FUNCTION_BLOCK FB_IEDClient IMPLEMENTS I_ScsmAbortIndEventSink, I_ScsmGetServerDirectoryCnfEventSink, I_ScsmGetLogicalDeviceDirectoryCnfEventSink, I_ScsmGetLogicalNodeDirectoryCnfEventSink, I_ScsmGetDataValuesCnfEventSink, I_ScsmSetDataValuesCnfEventSink, I_ScsmReportIndEventSink, I_ScsmControlCnfEventSink, I_ScsmLastApplErrorIndEventSink, I_ScsmCommandTerminationIndEventSink
VAR_INPUT
	fbConnection		: FB_iec61850ClientClass := (ipAbortInd:=THIS^, ipGetServerDirectoryCnf:=THIS^, ipGetLogicalDeviceDirectoryCnf:=THIS^, ipGetLogicalNodeDirectoryCnf:=THIS^, ipGetDataValuesCnf:=THIS^, ipSetDataValuesCnf:=THIS^, ipReportInd:=THIS^, ipControlCnf:=THIS^, ipLastApplErrorInd:=THIS^, ipCommandTerminationInd:=THIS^);
END_VAR
VAR
	_bAbort				: BOOL; (* Rising edge activates AbortReq() command execution *)
	_bDisconnect		: BOOL; (* Rising edge activates ReleaseReq() command execution *)
	_bConnect			: BOOL; (* Rising edge activates AssociateReq() command execution *)
	_bReconnect			: BOOL := TRUE; (* TRUE => reconnect automatically *)
	_bReadAllData		: BOOL := TRUE; (* TRUE => read/refresh all data values on reconnect *)
	
	state				: BYTE;
	eState				: E_AsyncEnvironmentState; (* Environment state *)
	bBusy				: BOOL; (* If TRUE => command execution is busy *)
	bSuccess			: BOOL;
	ipResult			: I_AsyncServiceResultClass;
	sLastErrorResult	: T_MaxString;
	fbAbortReason		: FB_ServiceErrorClass := (stError:=SUCCESS_EVENT);
	sLastAbortReason	: T_MaxString;
	nInvokeID			: UDINT;
	eServiceError		: E_AcsiServiceError; (* Latest OnXyzCnf() or OnXyzInd() event handler error *)
	nServiceError		: UDINT; (* Counts OnXyzCnf() and OnXyzInd() event handler errors *)
	nCmdError			: UDINT; (* Counts xyzReq() command errors *)
	sObjReference		: T_AcsiObjectReference; (* DATA object reference *)
	sCtrlReference		: T_AcsiObjectReference; (* CONTROLLABLE-DATA object reference *)
	
	bGetServerDirectory				: BOOL := TRUE; (* Rising edge enumerates logical-devices *)
	bGetLogicalDeviceDirectory		: BOOL := TRUE; (* Rising edge enumerates logical-nodes *)
	bGetLogicalNodeDirectory		: BOOL := TRUE; (* Rising edge enumerates "IEDLD1/LLN0" data-sets *)
	bGetAllServerValues				: BOOL := TRUE; (* Rising edge reads all "IEDLD1" data attribute values *)
	bGetAllDataValues_LLN0_ST		: BOOL := TRUE; (* Rising edge reads all "IEDLD1/LLN0.ST" data attribute values (having selected functional constraint) *)
	bGetDataValues_LLN0_ST_Beh		: BOOL := TRUE; (* Rising edge reads all "IEDLD1/LLN0.ST.Beh" data attribute values (having selected functional constraint) *)

	bSetAllDataValues_LPHD1_DC							: BOOL := TRUE; (* Rising edge writes all "IEDLD1/LPHD1.DC" data attribute values (having selected functional constraint) *)
	bSetAllDataValues_LLN0_DC							: BOOL := TRUE; (* Rising edge writes all "IEDLD1/LLN0.DC" data attribute values (having selected functional constraint) *)
	bSetAllDataValues_MMXU1_DC							: BOOL := TRUE; (* Rising edge writes all "IEDLD1/MMXU1.DC" data attribute values (having selected functional constraint) *)
	bSetAllDataValues_XCBR1_DC							: BOOL := TRUE; (* Rising edge writes all "IEDLD1/XCBR1.DC" data attribute values (having selected functional constraint) *)
	bSetAllDataValues_CSWI1_DC							: BOOL := TRUE; (* Rising edge writes all "IEDLD1/CSWI1.DC" data attribute values (having selected functional constraint) *)
	bSetAllDataValues_LEDGGIO1_DC						: BOOL := TRUE; (* Rising edge writes all "IEDLD1/LEDGGIO1.DC" data attribute values (having selected functional constraint) *)
	bSetAllDataValues_LEDGGIO2_DC						: BOOL := TRUE; (* Rising edge writes all "IEDLD1/LEDGGIO2.DC" data attribute values (having selected functional constraint) *)
	bSetAllDataValues_LEDGGIO3_DC						: BOOL := TRUE; (* Rising edge writes all "IEDLD1/LEDGGIO3.DC" data attribute values (having selected functional constraint) *)
	bSetAllDataValues_LEDGGIO4_DC						: BOOL := TRUE; (* Rising edge writes all "IEDLD1/LEDGGIO4.DC" data attribute values (having selected functional constraint) *)
	bSetAllDataValues_LEDGGIO5_DC						: BOOL := TRUE; (* Rising edge writes all "IEDLD1/LEDGGIO5.DC" data attribute values (having selected functional constraint) *)
	bSetAllDataValues_LEDGGIO6_DC						: BOOL := TRUE; (* Rising edge writes all "IEDLD1/LEDGGIO6.DC" data attribute values (having selected functional constraint) *)
	bSetAllDataValues_LEDGGIO7_DC						: BOOL := TRUE; (* Rising edge writes all "IEDLD1/LEDGGIO7.DC" data attribute values (having selected functional constraint) *)
	bSetAllDataValues_LEDGGIO8_DC						: BOOL := TRUE; (* Rising edge writes all "IEDLD1/LEDGGIO8.DC" data attribute values (having selected functional constraint) *)

	bSetDataValues_MMXU1_CF_TotW						: BOOL := FALSE; (* Rising edge writes all "IEDLD1/MMXU1.CF.TotW" data attribute values (having selected functional constraint) *)
	bSetDataValues_LEDGGIO1_CF_AnOut1_sboClass			: BOOL := FALSE; (* Rising edge writes all "IEDLD1/MMXU1.CF.AnOut1.sboClass" data attribute values (having selected functional constraint) *)
	bSetDataValues_LEDGGIO1_CF_AnOut1_ctlModel			: BOOL := FALSE; (* Rising edge writes all "IEDLD1/MMXU1.CF.AnOut1.ctlModel" data attribute values (having selected functional constraint) *)
	bSetDataValues_LEDGGIO1_CF_AnOut1_units				: BOOL := FALSE; (* Rising edge writes all "IEDLD1/MMXU1.CF.AnOut1.units" data attribute values (having selected functional constraint) *)
	bSetDataValues_LEDGGIO1_CF_AnOut1_units_SIUnit		: BOOL := FALSE; (* Rising edge writes all "IEDLD1/MMXU1.CF.AnOut1.units.SIUnit" data attribute values (having selected functional constraint) *)
	bSetDataValues_LEDGGIO1_CF_AnOut1_units_multiplier	: BOOL := FALSE; (* Rising edge writes all "IEDLD1/MMXU1.CF.AnOut1.units.multiplier" data attribute values (having selected functional constraint) *)

	sVendor 	: T_MaxString := 'MyCompany';
	sSerNum		: T_MaxString := '123456';
	sModel		: T_MaxString := 'My61850Model';
	sLocation	: T_MaxString := 'MyLocation';
	nRev		: UDINT := 1;
END_VAR

fbConnection.Execute();
eState:= fbConnection.eState;

CASE state OF
	0: (* Initial state *)
		IF _bAbort THEN (* Abort connection => execute AbortReq() command *)
			_bAbort:= FALSE;
			bSuccess:= fbConnection.AbortReq(ipReason:=fbAbortReason, ipSink:=0, ipResult=>ipResult);
			state:= SEL(bSuccess, 100, 1);
		ELSIF eState = E_AsyncEnvironmentState.Idle AND (_bConnect OR _bReconnect) THEN (* Open/establish connection => execute AssociateReq() command *)
			_bConnect:= FALSE;
			bGetAllServerValues:= SEL(_bReadAllData, bGetAllServerValues, TRUE);
			bSuccess:= fbConnection.AssociateReq(ipSink:=0, ipResult=>ipResult);
			state:= SEL(bSuccess, 100, 1);
		ELSIF eState = E_AsyncEnvironmentState.Established AND _bDisconnect THEN (* Close/release connection => execute ReleaseReq() command *)
			_bDisconnect:= FALSE;
			bSuccess:= fbConnection.ReleaseReq(ipSink:=0, ipResult=>ipResult);
			state:= SEL(bSuccess, 100, 1);
		ELSIF eState = E_AsyncEnvironmentState.Established THEN (* Connection established => exchange IED data *)
			state:= 10;
		END_IF
		_bConnect:= FALSE;
		_bDisconnect:= FALSE;
		(*==================================================================================================================================================================*)
	1: (* Wait for AbortReq() or ReleaseReq() or AssociateReq() command completion *)
		IF ipResult <> 0 THEN
			ipResult.Execute();
			IF NOT (bBusy:=ipResult.IsBusy()) THEN
				state:= SEL(ipResult.IsCompleted(), 100(* failed or aborted *), 0(* succeeded *));
			END_IF
		END_IF
		(*==================================================================================================================================================================*)
	10: (* Read/Write IED data *)
		IF bGetServerDirectory THEN (* Example => execute GetServerDirectoryReq() command *)
			bGetServerDirectory:= FALSE;
			bSuccess:= fbConnection.GetServerDirectoryReq(ipServer:=fbIED, eClass:=E_AcsiServerDirectoryClass.LogicalDevice, hUser:=0, ipSink:=0, nInvokeID=>nInvokeID, ipResult=>ipResult);
			state:= SEL(bSuccess, 100, 11);
		ELSIF bGetLogicalDeviceDirectory THEN (* Example => execute GetLogicalDeviceDirectoryReq() command *)
			bGetLogicalDeviceDirectory:= FALSE;
			bSuccess:= fbConnection.GetLogicalDeviceDirectoryReq(ipLogicalDevice:=fbIED.IEDLD1, hUser:=0, ipSink:=0, nInvokeID=>nInvokeID, ipResult=>ipResult);
			state:= SEL(bSuccess, 100, 11);
		ELSIF bGetLogicalNodeDirectory THEN (* Example => execute GetLogicalNodeDirectoryReq() command *)
			bGetLogicalNodeDirectory:= FALSE;
			bSuccess:= fbConnection.GetLogicalNodeDirectoryReq(ipLogicalNode:=fbIED.IEDLD1.LLN0, eClass:=E_AcsiLogicalNodeClass.DataSet, hUser:=0, ipSink:=0, nInvokeID=>nInvokeID, ipResult=>ipResult);
			state:= SEL(bSuccess, 100, 11);
		ELSIF bGetAllServerValues THEN (* Example => execute GetAllServerValues() command *)
			bGetAllServerValues:= FALSE;
			bSuccess:= fbConnection.GetAllServerValuesReq(ipServer:=fbIED, hUser:=0, ipSink:=0, nInvokeID=>nInvokeID, ipResult=>ipResult);
			state:= SEL(bSuccess, 100, 11);
		ELSIF bGetAllDataValues_LLN0_ST THEN (* Example => execute GetAllDataValuesReq() command *)
			bGetAllDataValues_LLN0_ST:= FALSE;
			bSuccess:= fbConnection.GetAllDataValuesReq(ipLogicalNode:=fbIED.IEDLD1.LLN0, eFc:=E_AcsiFc.ST_, hUser:=0, ipSink:=0, nInvokeID=>nInvokeID, ipResult=>ipResult);
			state:= SEL(bSuccess, 100, 11);
		ELSIF bGetDataValues_LLN0_ST_Beh THEN (* Example => execute GetDataValuesReq() command *)
			bGetDataValues_LLN0_ST_Beh:= FALSE;
			bSuccess:= fbConnection.GetDataValuesReq(ipData:=fbIED.IEDLD1.LLN0.Beh, eFc:=E_AcsiFc.ST_, hUser:=0, ipSink:=0, nInvokeID=>nInvokeID, ipResult=>ipResult);
		(*==================================================================================================================================================================*)
		ELSIF bSetAllDataValues_LPHD1_DC THEN(* Example => execute SetAllDataValuesReq() command *)
			bSetAllDataValues_LPHD1_DC:= FALSE;

			(* As example we modify some description data values *)
			nRev:= nRev + 1;
			fbIED.IEDLD1.LPHD1.PhyNam.Vendor.sValue:= sVendor;
			fbIED.IEDLD1.LPHD1.PhyNam.hwRev.sValue:= TO_STRING(TO_REAL(nRev));
			fbIED.IEDLD1.LPHD1.PhyNam.swRev.sValue:= TO_STRING(TO_REAL(nRev));
			fbIED.IEDLD1.LPHD1.PhyNam.serNum.sValue:= sSerNum;
			fbIED.IEDLD1.LPHD1.PhyNam.model.sValue:= sModel;
			fbIED.IEDLD1.LPHD1.PhyNam.location.sValue:= sLocation;
			
			bSuccess:= fbConnection.SetAllDataValuesReq(ipLogicalNode:=fbIED.IEDLD1.LPHD1, eFc:=E_AcsiFc.DC, hUser:=0, ipSink:=0, nInvokeID=>nInvokeID, ipResult=>ipResult); 
			state:= SEL(bSuccess, 100, 11);
		ELSIF bSetAllDataValues_LLN0_DC THEN(* Example => execute SetAllDataValuesReq() command *)
			bSetAllDataValues_LLN0_DC :=FALSE;

			(* As example we modify some description data values *)
			nRev:= nRev + 1;
			fbIED.IEDLD1.LLN0.NamPlt.vendor.sValue:= sVendor;
			fbIED.IEDLD1.LLN0.NamPlt.swRev.sValue:=  TO_STRING(TO_REAL(nRev));
			fbIED.IEDLD1.LLN0.NamPlt.d.sValue:= 'Demo of LLN0 node';
			fbIED.IEDLD1.LLN0.NamPlt.configRev.sValue:= TO_STRING(nRev);
			
			bSuccess:= fbConnection.SetAllDataValuesReq(ipLogicalNode:=fbIED.IEDLD1.LLN0, eFc:=E_AcsiFc.DC, hUser:=0, ipSink:=0, nInvokeID=>nInvokeID, ipResult=>ipResult); 
			state:= SEL(bSuccess, 100, 11);
		ELSIF bSetAllDataValues_MMXU1_DC THEN(* Example => execute SetAllDataValuesReq() command *)
			bSetAllDataValues_MMXU1_DC:= FALSE;

			(* As example we modify some description data values *)
			nRev:= nRev + 1;
			fbIED.IEDLD1.MMXU1.NamPlt.vendor.sValue:= sVendor;
			fbIED.IEDLD1.MMXU1.NamPlt.swRev.sValue:= TO_STRING(TO_REAL(nRev));
			fbIED.IEDLD1.MMXU1.NamPlt.d.sValue:= 'Demo of MMXU node';
			fbIED.IEDLD1.MMXU1.NamPlt.configRev.sValue:= TO_STRING(nRev);

			bSuccess:= fbConnection.SetAllDataValuesReq(ipLogicalNode:=fbIED.IEDLD1.MMXU1, eFc:=E_AcsiFc.DC, hUser:=0, ipSink:=0, nInvokeID=>nInvokeID, ipResult=>ipResult); 
			state:= SEL(bSuccess, 100, 11);
		ELSIF bSetAllDataValues_XCBR1_DC THEN(* Example => execute SetAllDataValuesReq() command *)
			bSetAllDataValues_XCBR1_DC:= FALSE;

			(* As example we modify some description data values *)
			nRev:= nRev + 1;
			fbIED.IEDLD1.XCBR1.NamPlt.vendor.sValue:= sVendor;
			fbIED.IEDLD1.XCBR1.NamPlt.swRev.sValue:= TO_STRING(TO_REAL(nRev));
			fbIED.IEDLD1.XCBR1.NamPlt.d.sValue:= 'Demo of XCBR1 node';
			fbIED.IEDLD1.XCBR1.NamPlt.configRev.sValue:= TO_STRING(nRev);

			bSuccess:= fbConnection.SetAllDataValuesReq(ipLogicalNode:=fbIED.IEDLD1.XCBR1, eFc:=E_AcsiFc.DC, hUser:=0, ipSink:=0, nInvokeID=>nInvokeID, ipResult=>ipResult); 
			state:= SEL(bSuccess, 100, 11);
		ELSIF bSetAllDataValues_CSWI1_DC THEN(* Example => execute SetAllDataValuesReq() command *)
			bSetAllDataValues_CSWI1_DC:= FALSE;

			(* As example we modify some description data values *)
			nRev:= nRev + 1;
			fbIED.IEDLD1.CSWI1.NamPlt.vendor.sValue:= sVendor;
			fbIED.IEDLD1.CSWI1.NamPlt.swRev.sValue:= TO_STRING(TO_REAL(nRev));
			fbIED.IEDLD1.CSWI1.NamPlt.d.sValue:= 'Demo of CSWI node';
			fbIED.IEDLD1.CSWI1.NamPlt.configRev.sValue:= TO_STRING(nRev);

			bSuccess:= fbConnection.SetAllDataValuesReq(ipLogicalNode:=fbIED.IEDLD1.CSWI1, eFc:=E_AcsiFc.DC, hUser:=0, ipSink:=0, nInvokeID=>nInvokeID, ipResult=>ipResult); 
			state:= SEL(bSuccess, 100, 11);
		ELSIF bSetAllDataValues_LEDGGIO1_DC THEN(* Example => execute SetAllDataValuesReq() command *)
			bSetAllDataValues_LEDGGIO1_DC:= FALSE;

			(* As example we modify some description data values *)
			nRev:= nRev + 1;
			fbIED.IEDLD1.LEDGGIO1.NamPlt.vendor.sValue:= sVendor;
			fbIED.IEDLD1.LEDGGIO1.NamPlt.swRev.sValue:= TO_STRING(TO_REAL(nRev));
			fbIED.IEDLD1.LEDGGIO1.NamPlt.d.sValue:= 'Demo of LEDGGIO1 node';

			bSuccess:= fbConnection.SetAllDataValuesReq(ipLogicalNode:=fbIED.IEDLD1.LEDGGIO1, eFc:=E_AcsiFc.DC, hUser:=0, ipSink:=0, nInvokeID=>nInvokeID, ipResult=>ipResult); 
			state:= SEL(bSuccess, 100, 11);
		ELSIF bSetAllDataValues_LEDGGIO2_DC THEN(* Example => execute SetAllDataValuesReq() command *)
			bSetAllDataValues_LEDGGIO2_DC:= FALSE;

			(* As example we modify some description data values *)
			nRev:= nRev + 1;
			fbIED.IEDLD1.LEDGGIO2.NamPlt.vendor.sValue:= sVendor;
			fbIED.IEDLD1.LEDGGIO2.NamPlt.swRev.sValue:= TO_STRING(TO_REAL(nRev));
			fbIED.IEDLD1.LEDGGIO2.NamPlt.d.sValue:= 'Demo of LEDGGIO2 node';

			bSuccess:= fbConnection.SetAllDataValuesReq(ipLogicalNode:=fbIED.IEDLD1.LEDGGIO2, eFc:=E_AcsiFc.DC, hUser:=0, ipSink:=0, nInvokeID=>nInvokeID, ipResult=>ipResult); 
			state:= SEL(bSuccess, 100, 11);
		ELSIF bSetAllDataValues_LEDGGIO3_DC THEN(* Example => execute SetAllDataValuesReq() command *)
			bSetAllDataValues_LEDGGIO3_DC:= FALSE;

			(* As example we modify some description data values *)
			nRev:= nRev + 1;
			fbIED.IEDLD1.LEDGGIO3.NamPlt.vendor.sValue:= sVendor;
			fbIED.IEDLD1.LEDGGIO3.NamPlt.swRev.sValue:= TO_STRING(TO_REAL(nRev));
			fbIED.IEDLD1.LEDGGIO3.NamPlt.d.sValue:= 'Demo of LEDGGIO3 node';

			bSuccess:= fbConnection.SetAllDataValuesReq(ipLogicalNode:=fbIED.IEDLD1.LEDGGIO3, eFc:=E_AcsiFc.DC, hUser:=0, ipSink:=0, nInvokeID=>nInvokeID, ipResult=>ipResult); 
			state:= SEL(bSuccess, 100, 11);
		ELSIF bSetAllDataValues_LEDGGIO4_DC THEN(* Example => execute SetAllDataValuesReq() command *)
			bSetAllDataValues_LEDGGIO4_DC:= FALSE;

			(* As example we modify some description data values *)
			nRev:= nRev + 1;
			fbIED.IEDLD1.LEDGGIO4.NamPlt.vendor.sValue:= sVendor;
			fbIED.IEDLD1.LEDGGIO4.NamPlt.swRev.sValue:= TO_STRING(TO_REAL(nRev));
			fbIED.IEDLD1.LEDGGIO4.NamPlt.d.sValue:= 'Demo of LEDGGIO4 node';

			bSuccess:= fbConnection.SetAllDataValuesReq(ipLogicalNode:=fbIED.IEDLD1.LEDGGIO4, eFc:=E_AcsiFc.DC, hUser:=0, ipSink:=0, nInvokeID=>nInvokeID, ipResult=>ipResult); 
			state:= SEL(bSuccess, 100, 11);
		ELSIF bSetAllDataValues_LEDGGIO5_DC THEN(* Example => execute SetAllDataValuesReq() command *)
			bSetAllDataValues_LEDGGIO5_DC:= FALSE;

			(* As example we modify some description data values *)
			nRev:= nRev + 1;
			fbIED.IEDLD1.LEDGGIO5.NamPlt.vendor.sValue:= sVendor;
			fbIED.IEDLD1.LEDGGIO5.NamPlt.swRev.sValue:= TO_STRING(TO_REAL(nRev));
			fbIED.IEDLD1.LEDGGIO5.NamPlt.d.sValue:= 'Demo of LEDGGIO5 node';

			bSuccess:= fbConnection.SetAllDataValuesReq(ipLogicalNode:=fbIED.IEDLD1.LEDGGIO5, eFc:=E_AcsiFc.DC, hUser:=0, ipSink:=0, nInvokeID=>nInvokeID, ipResult=>ipResult); 
			state:= SEL(bSuccess, 100, 11);
		ELSIF bSetAllDataValues_LEDGGIO6_DC THEN(* Example => execute SetAllDataValuesReq() command *)
			bSetAllDataValues_LEDGGIO6_DC:= FALSE;

			(* As example we modify some description data values *)
			nRev:= nRev + 1;
			fbIED.IEDLD1.LEDGGIO6.NamPlt.vendor.sValue:= sVendor;
			fbIED.IEDLD1.LEDGGIO6.NamPlt.swRev.sValue:= TO_STRING(TO_REAL(nRev));
			fbIED.IEDLD1.LEDGGIO6.NamPlt.d.sValue:= 'Demo of LEDGGIO6 node';

			bSuccess:= fbConnection.SetAllDataValuesReq(ipLogicalNode:=fbIED.IEDLD1.LEDGGIO6, eFc:=E_AcsiFc.DC, hUser:=0, ipSink:=0, nInvokeID=>nInvokeID, ipResult=>ipResult); 
			state:= SEL(bSuccess, 100, 11);
		ELSIF bSetAllDataValues_LEDGGIO7_DC THEN(* Example => execute SetAllDataValuesReq() command *)
			bSetAllDataValues_LEDGGIO7_DC:= FALSE;

			(* As example we modify some description data values *)
			nRev:= nRev + 1;
			fbIED.IEDLD1.LEDGGIO7.NamPlt.vendor.sValue:= sVendor;
			fbIED.IEDLD1.LEDGGIO7.NamPlt.swRev.sValue:= TO_STRING(TO_REAL(nRev));
			fbIED.IEDLD1.LEDGGIO7.NamPlt.d.sValue:= 'Demo of LEDGGIO7 node';

			bSuccess:= fbConnection.SetAllDataValuesReq(ipLogicalNode:=fbIED.IEDLD1.LEDGGIO7, eFc:=E_AcsiFc.DC, hUser:=0, ipSink:=0, nInvokeID=>nInvokeID, ipResult=>ipResult); 
			state:= SEL(bSuccess, 100, 11);
		ELSIF bSetAllDataValues_LEDGGIO8_DC THEN(* Example => execute SetAllDataValuesReq() command *)
			bSetAllDataValues_LEDGGIO8_DC:= FALSE;

			(* As example we modify some description data values *)
			nRev:=nRev + 1;
			fbIED.IEDLD1.LEDGGIO8.NamPlt.vendor.sValue:= sVendor;
			fbIED.IEDLD1.LEDGGIO8.NamPlt.swRev.sValue:= TO_STRING(TO_REAL(nRev));
			fbIED.IEDLD1.LEDGGIO8.NamPlt.d.sValue:= 'Demo of LEDGGIO8 node';

			bSuccess:= fbConnection.SetAllDataValuesReq(ipLogicalNode:=fbIED.IEDLD1.LEDGGIO8, eFc:=E_AcsiFc.DC, hUser:=0, ipSink:=0, nInvokeID=>nInvokeID, ipResult=>ipResult); 
			state:= SEL(bSuccess, 100, 11);
		(*==================================================================================================================================================================*)
		ELSIF bSetDataValues_MMXU1_CF_TotW THEN(* Example => execute SetDataValuesReq() command *)
			bSetDataValues_MMXU1_CF_TotW:= FALSE;
			fbIED.IEDLD1.MMXU1.TotW.units.SIUnit.eValue:= SEL(fbIED.IEDLD1.MMXU1.TotW.units.SIUnit.eValue = E_AcsiSIUnit.Volt, E_AcsiSIUnit.Volt, E_AcsiSIUnit.Watt);
 			fbIED.IEDLD1.MMXU1.TotW.units.multiplier.eValue:= SEL(fbIED.IEDLD1.MMXU1.TotW.units.multiplier.eValue = E_AcsiMultiplier.Milli, E_AcsiMultiplier.Milli, E_AcsiMultiplier.Kilo);

 			fbIED.IEDLD1.MMXU1.TotW.db.nValue:= SEL(fbIED.IEDLD1.MMXU1.TotW.db.nValue = 0, 0, 1000);
 			fbIED.IEDLD1.MMXU1.TotW.zeroDb.nValue:= SEL(fbIED.IEDLD1.MMXU1.TotW.zeroDb.nValue = 0, 0, 1000);
 			fbIED.IEDLD1.MMXU1.TotW.sVC.scaleFactor.fValue:= SEL(fbIED.IEDLD1.MMXU1.TotW.sVC.scaleFactor.fValue = 0.0, 0.0, 2.0);
 			fbIED.IEDLD1.MMXU1.TotW.sVC.offset.fValue:= SEL(fbIED.IEDLD1.MMXU1.TotW.sVC.offset.fValue = 0.0, 0.0, 10.0);
			
			bSuccess:= fbConnection.SetDataValuesReq(ipData:=fbIED.IEDLD1.MMXU1.TotW, eFc:=E_AcsiFc.CF, hUser:=0, ipSink:=0, nInvokeID=>nInvokeID, ipResult=>ipResult); 
			state:= SEL(bSuccess, 100, 11);
		(*==================================================================================================================================================================*)
		ELSIF bSetDataValues_LEDGGIO1_CF_AnOut1_sboClass THEN(* Example => execute SetDataValuesReq() command *)
			bSetDataValues_LEDGGIO1_CF_AnOut1_sboClass:= FALSE;
			fbIED.IEDLD1.LEDGGIO1.AnOut1.sboClass.eValue:= SEL(fbIED.IEDLD1.LEDGGIO1.AnOut1.sboClass.eValue = E_AcsiSboClasses.OperateOnce, E_AcsiSboClasses.OperateOnce, E_AcsiSboClasses.OperateMany);
			bSuccess:= fbConnection.SetDataValuesReq(ipData:=fbIED.IEDLD1.LEDGGIO1.AnOut1.sboClass, eFc:=E_AcsiFc.CF, hUser:=0, ipSink:=0, nInvokeID=>nInvokeID, ipResult=>ipResult); 
			state:= SEL(bSuccess, 100, 11);
		(*==================================================================================================================================================================*)
		ELSIF bSetDataValues_LEDGGIO1_CF_AnOut1_ctlModel THEN(* Example => execute SetDataValuesReq() command *)
			bSetDataValues_LEDGGIO1_CF_AnOut1_ctlModel:= FALSE;
			fbIED.IEDLD1.LEDGGIO1.AnOut1.ctlModel.eValue:= SEL(fbIED.IEDLD1.LEDGGIO1.AnOut1.ctlModel.eValue = E_AcsiCtlModels.SBOWithEnhancedSecurity, E_AcsiCtlModels.SBOWithEnhancedSecurity, E_AcsiCtlModels.DirectWithNormalSecurity);
			bSuccess:= fbConnection.SetDataValuesReq(ipData:=fbIED.IEDLD1.LEDGGIO1.AnOut1.ctlModel, eFc:=E_AcsiFc.CF, hUser:=0, ipSink:=0, nInvokeID=>nInvokeID, ipResult=>ipResult); 
			state:= SEL(bSuccess, 100, 11);
		(*==================================================================================================================================================================*)
		ELSIF bSetDataValues_LEDGGIO1_CF_AnOut1_units THEN(* Example => execute SetDataValuesReq() command *)
			bSetDataValues_LEDGGIO1_CF_AnOut1_units:= FALSE;
			fbIED.IEDLD1.LEDGGIO1.AnOut1.units.SIUnit.eValue:= SEL(fbIED.IEDLD1.LEDGGIO1.AnOut1.units.SIUnit.eValue = E_AcsiSIUnit.Volt, E_AcsiSIUnit.Volt, E_AcsiSIUnit.Ampere);
 			fbIED.IEDLD1.LEDGGIO1.AnOut1.units.multiplier.eValue:= SEL(fbIED.IEDLD1.LEDGGIO1.AnOut1.units.multiplier.eValue = E_AcsiMultiplier.Milli, E_AcsiMultiplier.Milli, E_AcsiMultiplier.Kilo);
			bSuccess:= fbConnection.SetDataValuesReq(ipData:=fbIED.IEDLD1.LEDGGIO1.AnOut1.units, eFc:=E_AcsiFc.CF, hUser:=0, ipSink:=0, nInvokeID=>nInvokeID, ipResult=>ipResult); 
			state:= SEL(bSuccess, 100, 11);
		(*==================================================================================================================================================================*)
		ELSIF bSetDataValues_LEDGGIO1_CF_AnOut1_units_SIUnit THEN(* Example => execute SetDataValuesReq() command *)
			bSetDataValues_LEDGGIO1_CF_AnOut1_units_SIUnit:= FALSE;
			fbIED.IEDLD1.LEDGGIO1.AnOut1.units.SIUnit.eValue:= SEL(fbIED.IEDLD1.LEDGGIO1.AnOut1.units.SIUnit.eValue = E_AcsiSIUnit.Volt, E_AcsiSIUnit.Volt, E_AcsiSIUnit.Ampere);
			bSuccess:= fbConnection.SetDataValuesReq(ipData:=fbIED.IEDLD1.LEDGGIO1.AnOut1.units.SIUnit, eFc:=E_AcsiFc.CF, hUser:=0, ipSink:=0, nInvokeID=>nInvokeID, ipResult=>ipResult); 
			state:= SEL(bSuccess, 100, 11);
		(*==================================================================================================================================================================*)
		ELSIF bSetDataValues_LEDGGIO1_CF_AnOut1_units_multiplier THEN(* Example => execute SetDataValuesReq() command *)
			bSetDataValues_LEDGGIO1_CF_AnOut1_units_multiplier:= FALSE;
 			fbIED.IEDLD1.LEDGGIO1.AnOut1.units.multiplier.eValue:= SEL(fbIED.IEDLD1.LEDGGIO1.AnOut1.units.multiplier.eValue = E_AcsiMultiplier.Milli, E_AcsiMultiplier.Milli, E_AcsiMultiplier.Kilo);
			bSuccess:= fbConnection.SetDataValuesReq(ipData:=fbIED.IEDLD1.LEDGGIO1.AnOut1.units.multiplier, eFc:=E_AcsiFc.CF, hUser:=0, ipSink:=0, nInvokeID=>nInvokeID, ipResult=>ipResult); 
			state:= SEL(bSuccess, 100, 11);
		ELSE
			state:= 0;
		END_IF
		(*==================================================================================================================================================================*)
	11: (* Wait for GetServerDirectoryReq(), GetLogicalDeviceDirectoryReq(), GetLogicalNodeDirectoryReq(), GetAllServerValuesReq(), GetAllDataValuesReq() or GetDataValuesReq() or SetAllDataValuesReq() or SetDataValuesReq() command completion *)
		IF ipResult <> 0 THEN
			ipResult.Execute();
			IF NOT (bBusy:=ipResult.IsBusy()) THEN
				state:= SEL(ipResult.IsCompleted(), 100(* failed or aborted *), 0(* succeeded *));
			END_IF
		END_IF
		(*==================================================================================================================================================================*)
	100: (* Error state *)
		state:= 0;
		IF ipResult <> 0 THEN
			nCmdError:= nCmdError + 1;
			sLastErrorResult:= ipResult.Dump();
		END_IF
END_CASE

PROPERTY bAbort : BOOL
SET
_bAbort:= bAbort;
END_SET
END_PROPERTY

PROPERTY bConnect : BOOL
SET
_bConnect:= bConnect;
END_SET
END_PROPERTY

PROPERTY bDisconnect : BOOL
SET
_bDisconnect:= bDisconnect;
END_SET
END_PROPERTY

PROPERTY bReconnect : BOOL
SET
_bReconnect:= bReconnect;
END_SET
END_PROPERTY

(* This method receives IEC61850::Abort.ind primitive. *)
METHOD OnAbortInd
VAR_INPUT
	ipAA		: I_ScsmAssociationClass; (* Application association. If = 0 => optional. *)
	bPAbort		: BOOL; (* TRUE => P-Abort.request(), issued by provider, FALSE => Abort.request(), issued by user. *)
	ipReason	: I_ServiceErrorClass; (* Abort reason. *)
	ipData		: I_BaseStreamClass; (* Optional data. If = 0 => default, no data. *)
END_VAR
VAR
END_VAR
IF ipReason <> 0 THEN
	sLastAbortReason:= ipReason.Dump();
END_IF
END_METHOD

(* This method receives buffered IEC61850::Report.ind primitive. *)
METHOD OnBufferedReportInd
VAR_INPUT
	ipAA		: I_ScsmAssociationClass; (* Application association. If = 0 => optional. *)
	info		: ST_ScsmReportEventInfo;
	ipBrcb		: I_AcsiCommonBufferedReportControlBlockClass; (* Interface pointer to BRCB object. *)
	ipDataSet	: I_AcsiCommonDataSetClass; (* Interface pointer to data-set object. *)
	ipData		: I_AcsiCommonDataClass; (* Interface pointer to reported data object. *)
	eFc			: E_AcsiFc; (* Functional constraint of reported data. *)
	eError		: E_AcsiServiceError; (* Data access error code. *)
END_VAR
VAR
END_VAR
IF eError <> E_AcsiServiceError.NoError THEN
	eServiceError:= eError;
	nServiceError:= nServiceError + 1;
END_IF
IF ipData <> 0 THEN
	sObjReference:= ipData.GetObjectReference();
END_IF
END_METHOD

(* This method receives IEC61850::CommandTermination.ind primitive. *)
METHOD OnCommandTerminationInd
VAR_INPUT
	ipAA		: I_ScsmAssociationClass; (* Application association. If = 0 => optional. *)
	info		: ST_ScsmCommandTerminationEventInfo;
	ipCtrl		: I_AcsiCommonControllableDataClass; (* Interface pointer to controllable data object. *)
	ipData		: I_AcsiCommonDataClass; (* Interface pointer to Oper/Cancel/SBO or SBOw data object. *)
	eFc			: E_AcsiFc; (* Functional constraint (CO). *)
	eError		: E_AcsiServiceError; (* Error code. *)
END_VAR
VAR
END_VAR
IF eError <> E_AcsiServiceError.NoError THEN
	eServiceError:= eError;
	nServiceError:= nServiceError + 1;
END_IF
IF ipCtrl <> 0 THEN
	sCtrlReference:= ipCtrl.GetObjectReference();
END_IF
IF ipData <> 0 THEN
	sObjReference:= ipData.GetObjectReference();
END_IF
END_METHOD

(* This method receives IEC61850::Control[Select|Operate|SelectWithValue|Cancel].cnf primitive. *)
METHOD OnControlCnf
VAR_INPUT
	ipAA		: I_ScsmAssociationClass; (* Application association. If = 0 => optional. *)
	info		: ST_ScsmConfirmedEventInfo;
	ipCtrl		: I_AcsiCommonControllableDataClass; (* Interface pointer to controllable data object. *)
	ipData		: I_AcsiCommonDataClass; (* Interface pointer to Oper/Cancel/SBO or SBOw data object. *)
	eFc			: E_AcsiFc; (* Functional constraint (CO). *)
	eError		: E_AcsiServiceError; (* Write/Read data access error code. *)
END_VAR
VAR
END_VAR
IF eError <> E_AcsiServiceError.NoError THEN
	eServiceError:= eError;
	nServiceError:= nServiceError + 1;
END_IF
IF ipCtrl <> 0 THEN
	sCtrlReference:= ipCtrl.GetObjectReference();
END_IF
IF ipData <> 0 THEN
	sObjReference:= ipData.GetObjectReference();
END_IF
END_METHOD

(* This method receives IEC61850::GetDataValues.cnf primitive. *)
METHOD OnGetDataValuesCnf
VAR_INPUT
	ipAA		: I_ScsmAssociationClass; (* Application association. If = 0 => optional. *)
	info		: ST_ScsmConfirmedEventInfo;
	ipData		: I_AcsiCommonDataClass; (* Interface pointer to read data object. *)
	eFc			: E_AcsiFc; (* Functional constraint of read data. *)
	eError		: E_AcsiServiceError; (* Data access error code. *)
END_VAR
VAR
END_VAR
IF eError <> E_AcsiServiceError.NoError THEN
	eServiceError:= eError;
	nServiceError:= nServiceError + 1;
END_IF
IF ipData <> 0 THEN
	sObjReference:= ipData.GetObjectReference();
END_IF
END_METHOD

(* This method receives IEC61850::GetLogicalDeviceDirectory.cnf primitive. *)
METHOD OnGetLogicalDeviceDirectoryCnf
VAR_INPUT
	ipAA				: I_ScsmAssociationClass; (* Application association. If = 0 => optional. *)
	info				: ST_ScsmConfirmedEventInfo;
	ipLogicalDevice		: I_AcsiCommonLogicalDeviceClass; (* Interface pointer to logical-device object. *)
	sObjectReference	: T_AcsiObjectReference;
	eError				: E_AcsiServiceError; (* Logical-device class access error code. *)
END_VAR
VAR
END_VAR
IF eError <> E_AcsiServiceError.NoError THEN
	eServiceError:= eError;
	nServiceError:= nServiceError + 1;
END_IF
sObjReference:= sObjectReference;
END_METHOD

(* This method receives IEC61850::GetLogicalNodeDirectory.cnf primitive. *)
METHOD OnGetLogicalNodeDirectoryCnf
VAR_INPUT
	ipAA				: I_ScsmAssociationClass; (* Application association. If = 0 => optional. *)
	info				: ST_ScsmConfirmedEventInfo;
	ipLogicalNode		: I_AcsiCommonLogicalNodeClass; (* Interface pointer to logical-node object. *)
	eClass				: E_AcsiLogicalNodeClass; (* Logical-node directory class (BRCB, URCB, DATA-SET, ... ). *)
	sObjectReference	: T_AcsiObjectReference;
	eError				: E_AcsiServiceError; (* Logical-node class access error code. *)
END_VAR
VAR
END_VAR
IF eError <> E_AcsiServiceError.NoError THEN
	eServiceError:= eError;
	nServiceError:= nServiceError + 1;
END_IF
sObjReference:= sObjectReference;
END_METHOD

(* This method receives IEC61850::GetServerDirectory.cnf primitive. *)
METHOD OnGetServerDirectoryCnf
VAR_INPUT
	ipAA				: I_ScsmAssociationClass; (* Application association. If = 0 => optional. *)
	info				: ST_ScsmConfirmedEventInfo;
	ipServer			: I_AcsiCommonIntelligentElectronicDeviceClass; (* Interface pointer to server object. *)
	eClass				: E_AcsiServerDirectoryClass; (* Server directory class (logical-device or file). *)
	sObjectReference	: T_AcsiObjectReference;
	eError				: E_AcsiServiceError; (* Server class (logical-device) access error code. *)
END_VAR
VAR
END_VAR
IF eError <> E_AcsiServiceError.NoError THEN
	eServiceError:= eError;
	nServiceError:= nServiceError + 1;
END_IF
sObjReference:= sObjectReference;
END_METHOD

(* This method receives IEC61850::LastApplError.ind primitive. *)
METHOD OnLastApplErrorInd
VAR_INPUT
	ipAA		: I_ScsmAssociationClass; (* Application association. If = 0 => optional. *)
	info		: ST_ScsmAdditionalCauseDiagnosticEventInfo;
	ipCtrl		: I_AcsiCommonControllableDataClass; (* Interface pointer to controllable data object. *)
	eError		: E_AcsiServiceError; (* Error code. *)
END_VAR
VAR
END_VAR
IF eError <> E_AcsiServiceError.NoError THEN
	eServiceError:= eError;
	nServiceError:= nServiceError + 1;
END_IF
IF ipCtrl <> 0 THEN
	sCtrlReference:= ipCtrl.GetObjectReference();
END_IF
END_METHOD

(* This method receives IEC61850::SetDataValues.cnf primitive. *)
METHOD OnSetDataValuesCnf
VAR_INPUT
	ipAA		: I_ScsmAssociationClass; (* Application association. If = 0 => optional. *)
	info		: ST_ScsmConfirmedEventInfo;
	ipData		: I_AcsiCommonDataClass; (* Interface pointer to written data object. *)
	eFc			: E_AcsiFc; (* Functional constraint of written data. *)
	eError		: E_AcsiServiceError; (* Data access error code. *)
END_VAR
VAR
END_VAR
IF eError <> E_AcsiServiceError.NoError THEN
	eServiceError:= eError;
	nServiceError:= nServiceError + 1;
END_IF
IF ipData <> 0 THEN
	sObjReference:= ipData.GetObjectReference();
END_IF
END_METHOD

(* This method receives unbuffered IEC61850::Report.ind primitive. *)
METHOD OnUnbufferedReportInd
VAR_INPUT
	ipAA		: I_ScsmAssociationClass; (* Application association. If = 0 => optional. *)
	info		: ST_ScsmReportEventInfo;
	ipUrcb		: I_AcsiCommonUnbufferedReportControlBlockClass; (* Interface pointer to URCB object. *)
	ipDataSet	: I_AcsiCommonDataSetClass; (* Interface pointer to dataset object. *)
	ipData		: I_AcsiCommonDataClass; (* Interface pointer to reported data object. *)
	eFc			: E_AcsiFc; (* Functional constraint of reported data. *)
	eError		: E_AcsiServiceError; (* Data access error code. *)
END_VAR
VAR
END_VAR
IF eError <> E_AcsiServiceError.NoError THEN
	eServiceError:= eError;
	nServiceError:= nServiceError + 1;
END_IF
IF ipData <> 0 THEN
	sObjReference:= ipData.GetObjectReference();
END_IF
END_METHOD

END_FUNCTION_BLOCK
